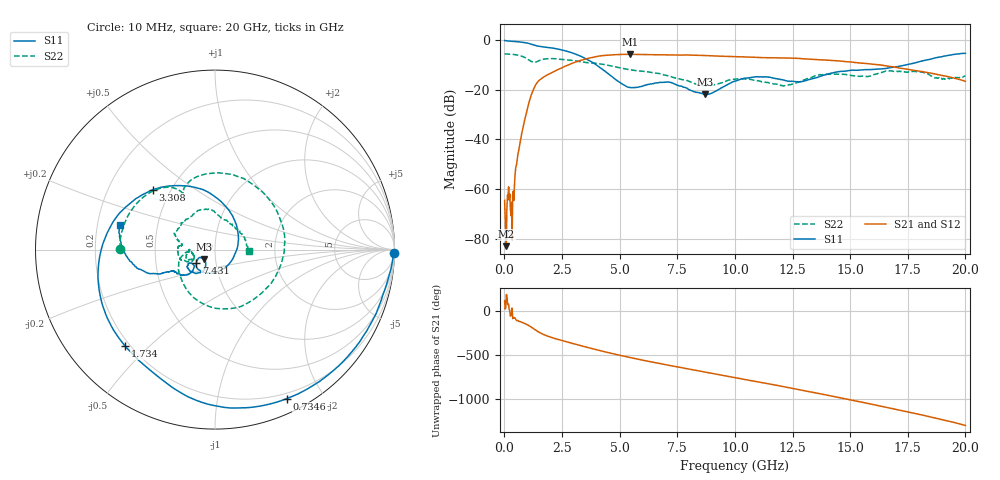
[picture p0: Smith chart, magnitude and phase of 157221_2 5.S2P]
!  2-Port S-parameters saved by WinCal
! VAR MeasName=S-Parameters (CALIBRATED_DATA) read from VNA (N5242A)
! VAR MeasDate=2015-5-26 16:47:34
! VAR NAME=157221_2 5
! VAR FILENAME=157221_2 5.S2P
! VAR DATE=2015-5-26 16:47:34
! VAR PHYS_PORTS=1,2
# Hz S DB R 50
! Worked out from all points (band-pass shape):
!   801 points, 10 MHz to 20 GHz, reference 50 ohm
!   highest |S21| = -5.63 dB at 5.457 GHz (marker M1); lowest = -83.1 dB at 84.96 MHz (marker M2)
!   |S21| within 3 dB of the highest: 3.118 GHz to 14.86 GHz (11.75 GHz wide, 131 % of centre); 14.89802 GHz to 14.90761 GHz (9.589 MHz wide, 0.0643 % of centre)
!   lowest |S11| = -21.8 dB at 8.706 GHz (marker M3), VSWR 1.18, Z = 43.9 - j4.64 ohm
!   |S11| at or under -10 dB: 4.003 GHz to 17.37 GHz (13.37 GHz wide, 125 % of centre)
!   |S22| runs from -18.4 to -5.5 dB; largest |S21 - S12| = 0.0094
!   S11 on the Smith chart (normalised r, x): 10 MHz: open; 734.6 MHz: 0.14, -1.58; 1.734 GHz: 0.18, -0.42; 3.308 GHz: 0.40, +0.35; 7.431 GHz: 0.80, -0.13; 20 GHz: 0.30, +0.12
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1e7  -0.04 -1.1  -64.53 117.1  -75.08 -124.8  -5.53 179.5
8.49625e7  -0.17 -8.6  -83.06 -172.1  -80.57 142.3  -5.51 175.3
2.099e8  -0.30 -19.4  -64.48 18.6  -63.42 20.1  -5.55 168.3
3.59825e8  -0.39 -32.4  -62.72 -85.3  -63.02 -84.8  -5.65 160.1
7.346375e8  -0.71 -64.2  -38.60 -125.1  -38.56 -125.3  -6.34 138.8
1.2094e9  -1.65 -101.9  -20.98 170.5  -20.95 170.3  -8.67 120.1
1.734138e9  -2.68 -132.9  -14.63 90.6  -14.60 90.4  -7.53 102.2
2.433788e9  -3.74 -174.1  -11.33 30.4  -11.31 30.0  -7.61 50.8
3.30835e9  -6.36 135.9  -8.08 -31.7  -8.10 -32.0  -8.62 -20.1
3.358325e9  -6.60 133.1  -7.92 -35.2  -7.94 -35.6  -8.67 -24.3
4.332838e9  -12.23 74.9  -6.09 -100.3  -6.11 -100.5  -9.75 -90.6
5.457275e9  -19.04 -22.4  -5.63 -167.7  -5.64 -167.8  -11.87 -135.2
6.681662e9  -17.08 -113.6  -5.80 127.6  -5.79 127.6  -13.36 -159.9
7.431288e9  -17.77 -143.6  -5.97 90.3  -5.93 90.0  -15.25 -172.0
8.70565e9  -21.80 -139.8  -6.12 26.9  -6.10 26.7  -18.21 -164.3
1.0005e10  -16.41 -121.9  -6.58 -35.6  -6.57 -36.1  -15.65 -159.8
1.152924e10  -14.88 -149.0  -6.99 -108.6  -6.99 -109.2  -17.27 -179.1
1.335332e10  -15.50 -136.9  -7.64 159.1  -7.60 158.8  -14.83 -160.5
1.477761e10  -12.41 -144.7  -8.56 84.6  -8.49 84.3  -13.73 175.0
1.667666e10  -11.13 -154.1  -10.46 -18.6  -10.44 -18.8  -12.29 158.3
1.805098e10  -8.46 -159.3  -12.48 -94.8  -12.47 -96.3  -12.76 102.0
2e10  -5.21 165.5  -16.52 142.1  -16.59 140.3  -14.48 -3.2
